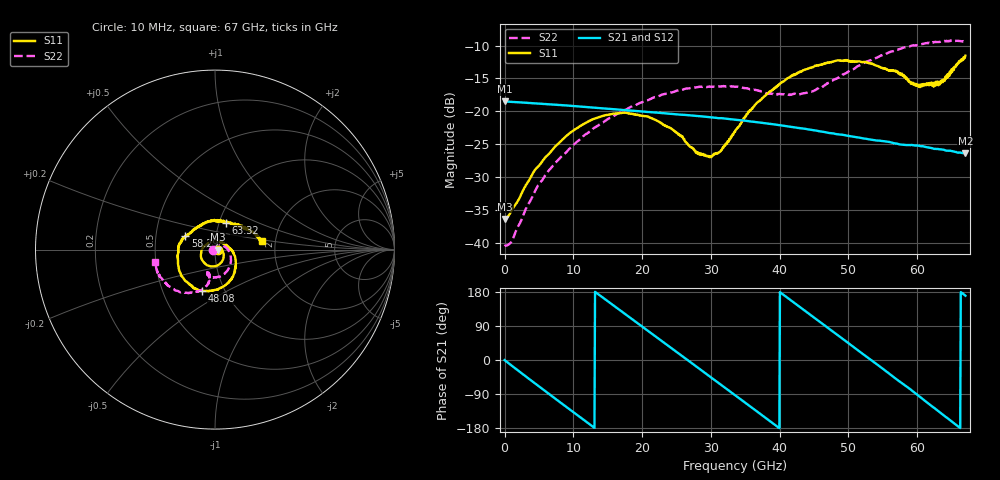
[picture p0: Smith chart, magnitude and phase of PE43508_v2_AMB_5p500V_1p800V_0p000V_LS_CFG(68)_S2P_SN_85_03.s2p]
!Keysight Technologies,N5227A,US51270237,A.10.43.00
!Date: Wednesday, August 22, 2018 17:13:42
!Correction: S11(Full 2 Port(1,3))
!S31(Full 2 Port(1,3))
!S13(Full 2 Port(1,3))
!S33(Full 2 Port(1,3))
!S2P File: Measurements: S11, S31, S13, S33:
# Hz S  dB  R 50
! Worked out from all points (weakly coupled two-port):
!   801 points, 10 MHz to 67 GHz, reference 50 ohm
!   highest |S21| = -18.48 dB at 10 MHz (marker M1); lowest = -26.4 dB at 67 GHz (marker M2)
!   lowest |S11| = -36.3 dB at 93.74 MHz (marker M3), VSWR 1.03, Z = 51.5 + j0.0237 ohm
!   |S11| at or under -10 dB: start of sweep to end of sweep
!   |S22| runs from -40.5 to -9.2 dB; largest |S21 - S12| = 0.00061
!   S11 on the Smith chart (normalised r, x): 10 MHz: 1.03, -0.00; 48.08 GHz: 0.78, -0.38; 58.29 GHz: 0.71, +0.11; 63.32 GHz: 1.07, +0.33; 67 GHz: 1.69, +0.18
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1e7  -36.26 -1.4  -18.48 -0.2  -18.48 -0.2  -40.49 -179.1
9.37375e7  -36.35 0.9  -18.49 -1.4  -18.51 -1.5  -40.40 175.8
1.01485e9  -35.13 8.4  -18.56 -14.5  -18.56 -14.5  -39.77 138.0
4.531825e9  -28.77 -1.6  -18.78 -63.2  -18.78 -63.2  -31.91 67.1
6.122838e9  -26.78 -14.9  -18.88 -85.0  -18.89 -84.9  -29.38 51.7
1.123082e10  -22.07 -62.7  -19.28 -154.2  -19.28 -154.2  -24.00 9.1
1.725992e10  -20.21 -115.4  -19.79 124.8  -19.79 124.9  -19.91 -28.5
2.236791e10  -21.52 -159.5  -20.22 56.5  -20.21 56.5  -17.70 -55.1
2.61361e10  -24.21 160.2  -20.53 6.2  -20.52 6.2  -16.61 -72.8
2.797832e10  -26.22 126.6  -20.70 -18.5  -20.71 -18.5  -16.34 -79.9
2.973681e10  -26.88 90.5  -20.87 -42.1  -20.86 -42.1  -16.21 -87.0
3.132782e10  -26.12 56.1  -21.03 -63.3  -21.04 -63.3  -16.20 -93.1
3.3505e10  -23.12 18.1  -21.26 -92.8  -21.27 -92.9  -16.25 -100.2
3.836178e10  -17.21 -32.7  -21.87 -158.2  -21.88 -158.2  -17.29 -108.6
4.472582e10  -13.32 -82.4  -22.81 115.7  -22.80 115.8  -16.97 -102.1
4.807532e10  -12.32 -107.5  -23.43 70.3  -23.42 70.3  -15.09 -100.8
5.251341e10  -12.53 -142.4  -24.15 10.2  -24.13 10.1  -12.49 -108.4
5.586291e10  -13.85 -176.1  -24.63 -35.4  -24.61 -35.8  -11.04 -120.5
5.82913e10  -14.83 155.3  -25.11 -68.0  -25.11 -68.3  -10.24 -129.8
6.004979e10  -15.88 126.2  -25.20 -92.3  -25.21 -92.7  -9.93 -137.2
6.331555e10  -15.88 68.6  -25.76 -138.4  -25.80 -139.0  -9.43 -151.8
6.7e10  -11.53 10.6  -26.35 169.7  -26.43 169.6  -9.29 -168.0
